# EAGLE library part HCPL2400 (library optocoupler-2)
HEWLETT PACKARD OPTO COUPLER
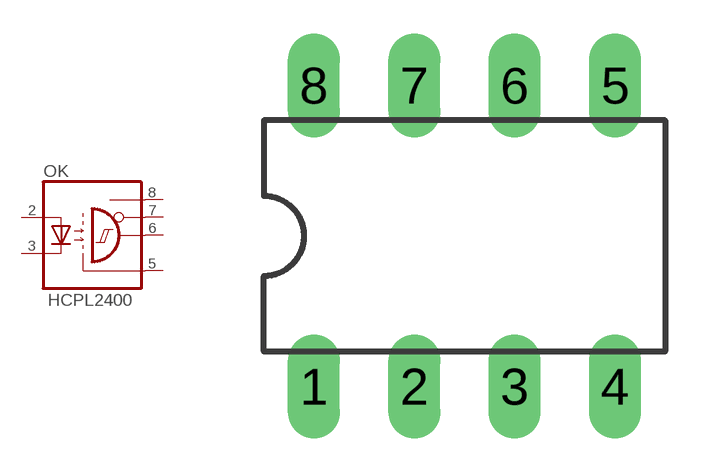
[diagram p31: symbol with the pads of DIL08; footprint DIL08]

Designator prefix OK

## HCPL2400  [DIL08]
2  A  pas
3  C  pas
5  GND  pas
6  VO  pas
7  VE  pas
8  VCC  pas

## Footprint DIL08 (pad centres in mm)
Dual In Line Package
drill 0.813 long: 1 -3.81,-3.81; 2 -1.27,-3.81; 3 1.27,-3.81; 4 3.81,-3.81; 5 3.81,3.81; 6 1.27,3.81; 7 -1.27,3.81; 8 -3.81,3.81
